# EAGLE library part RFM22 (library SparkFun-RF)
Hope RF RFM22 ISM Transciever Module The RFM22 is a low-power, low cost radio that is capable of operating in the 434MHz and 900MHz open bands. It's frequency is software defined and there are some very good libraries written for it. SparkFun Products SparkFun RFM22 Shield - 434MHz (DEV-11018)
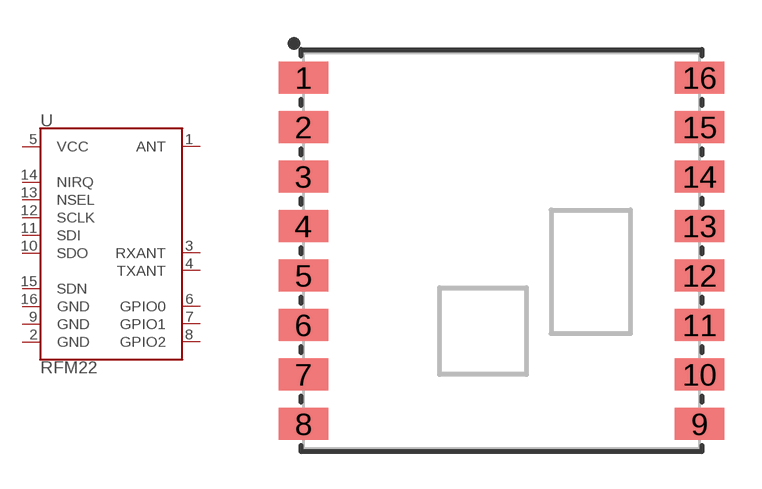
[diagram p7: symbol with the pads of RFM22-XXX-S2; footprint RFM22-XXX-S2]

Designator prefix -

## RFM22434MHZ (PROD_ID: IC-10007; SF_ID: WRL-10153; VALUE: 434MHz)  [RFM22-XXX-S2]
1  ANT
2  GND  pwr
3  RXANT  in
4  TXANT  in
5  VCC
6  GPIO0
7  GPIO1
8  GPIO2
9  GND  pwr
10  SDO  out
11  SDI  in
12  SCLK  in
13  NSEL  in
14  NIRQ  out
15  SDN  in
16  GND  pwr

## RFM22915MHZ (PROD_ID: IC-11750; SF_ID: WRL-12030; VALUE: 915MHz)  [RFM22-XXX-S2]
Pads as for RFM22-XXX-S2

## Footprint RFM22-XXX-S2 (pad centres in mm)
Hope RF RFM22 RF Transceiver Package for Hope RF s RFM22-xxx-S2 SMD wireless transciever, xxx is module s frequency band. SparkFun Link (915MHz) SparkFun Link (433 MHz) Datasheet
smd 2 x 1.3: 1 -8,7; 2 -8,5; 3 -8,3; 4 -8,1; 5 -8,-1; 6 -8,-3; 7 -8,-5; 8 -8,-7; 9 8,-7; 10 8,-5; 11 8,-3; 12 8,-1; 13 8,1; 14 8,3; 15 8,5; 16 8,7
